ORGANIZATION_BLOCK OB 81
TITLE = "Power Supply Fault"
AUTHOR : Esposito
FAMILY : EGAL_srl
NAME : PS_FLT
VERSION : 0.1


VAR_TEMP
  OB81_EV_CLASS : BYTE ;	//16#39, Event class 3, Entering event state, Internal fault event
  OB81_FLT_ID : BYTE ;	//16#XX, Fault identifcation code
  OB81_PRIORITY : BYTE ;	//26/28 (Priority of 1 is lowest)
  OB81_OB_NUMBR : BYTE ;	//81 (Organization block 81, OB81)
  OB81_RESERVED_1 : BYTE ;	//Reserved for system
  OB81_RESERVED_2 : BYTE ;	//Reserved for system
  OB81_MDL_ADDR : INT ;	//Reserved for system
  OB81_RESERVED_3 : BYTE ;	//Reserved for system
  OB81_RESERVED_4 : BYTE ;	//Reserved for system
  OB81_RESERVED_5 : BYTE ;	//Reserved for system
  OB81_RESERVED_6 : BYTE ;	//Reserved for system
  OB81_DATE_TIME : DATE_AND_TIME ;	//Date and time OB81 started
END_VAR
BEGIN
NETWORK
TITLE =BATTERY FAULT

      L     B#16#21;
      L     #OB81_FLT_ID;
      ==I   ;
      SPB   EAAH;
      L     B#16#22;
      <>I   ;
      R     DB102.DBX    1.0;
      BEB   ;
EAAH: S     DB102.DBX    1.0;
END_ORGANIZATION_BLOCK

